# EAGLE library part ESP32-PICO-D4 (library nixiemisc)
The ESP32-PICO-D4 is a System-in-Package (SIP) module that is based on ESP32, providing complete Wi-Fi and Bluetooth functionalities. The module has a size as small as 7.0±0.1 mm×7.0±0.1 mm×0.94±0.1 mm, thus requiring minimal PCB area. The module integrates a 4-MB SPI flash
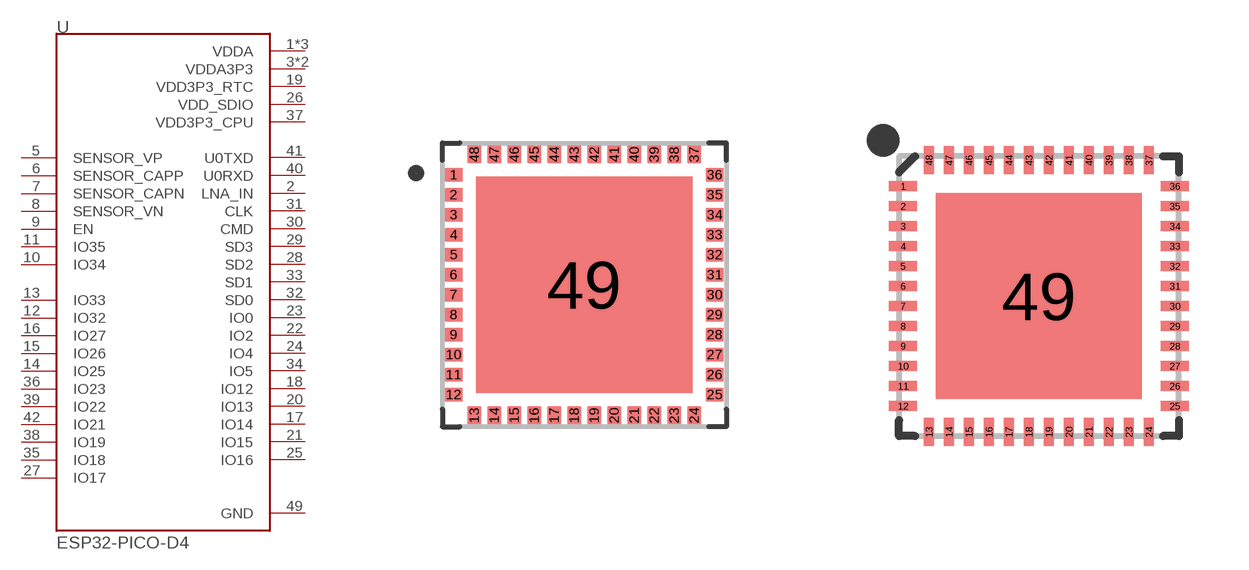
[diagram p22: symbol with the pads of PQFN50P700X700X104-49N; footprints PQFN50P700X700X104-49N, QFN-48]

Designator prefix U

## ESP32-PICO-D4 (AVAILABILITY: Unavailable; DESCRIPTION: WIFi/Bluetooth SIP; MF: Espressif Systems; MP: ESP32-PICO-D4; PACKAGE: SMD-48 Espressif Systems; PRICE: None)  [PQFN50P700X700X104-49N]
1  VDDA  pwr
2  LNA_IN
3  VDDA3P3  pwr
4  VDDA3P3  pwr
5  SENSOR_VP  in
6  SENSOR_CAPP  in
7  SENSOR_CAPN  in
8  SENSOR_VN  in
9  EN  in
10  IO34  in
11  IO35  in
12  IO32
13  IO33
14  IO25
15  IO26
16  IO27
17  IO14
18  IO12
19  VDD3P3_RTC  pwr
20  IO13
21  IO15
22  IO2
23  IO0
24  IO4
25  IO16
26  VDD_SDIO  pwr
27  IO17
28  SD2
29  SD3
30  CMD
31  CLK
32  SD0
33  SD1
34  IO5
35  IO18
36  IO23
37  VDD3P3_CPU  pwr
38  IO19
39  IO22
40  U0RXD
41  U0TXD
42  IO21
43  VDDA  pwr
46  VDDA  pwr
49  GND  pwr

## ESP32-PICO-D4QFN-48  [QFN-48]
Pads as for PQFN50P700X700X104-49N

## ESP32-PICO-D4QFN-48-7X7  [QFN48_7X7]
Pads as for PQFN50P700X700X104-49N

## Footprint PQFN50P700X700X104-49N (pad centres in mm)
smd 0.45 x 0.35: 1 -3.265,2.75; 2 -3.265,2.25; 3 -3.265,1.75; 4 -3.265,1.25; 5 -3.265,0.75; 6 -3.265,0.25; 7 -3.265,-0.25; 8 -3.265,-0.75; 9 -3.265,-1.25; 10 -3.265,-1.75; 11 -3.265,-2.25; 12 -3.265,-2.75; 25 3.265,-2.75; 26 3.265,-2.25; 27 3.265,-1.75; 28 3.265,-1.25; 29 3.265,-0.75; 30 3.265,-0.25; 31 3.265,0.25; 32 3.265,0.75; 33 3.265,1.25; 34 3.265,1.75; 35 3.265,2.25; 36 3.265,2.75
smd 0.35 x 0.45: 13 -2.75,-3.265; 14 -2.25,-3.265; 15 -1.75,-3.265; 16 -1.25,-3.265; 17 -0.75,-3.265; 18 -0.25,-3.265; 19 0.25,-3.265; 20 0.75,-3.265; 21 1.25,-3.265; 22 1.75,-3.265; 23 2.25,-3.265; 24 2.75,-3.265; 37 2.75,3.265; 38 2.25,3.265; 39 1.75,3.265; 40 1.25,3.265; 41 0.75,3.265; 42 0.25,3.265; 43 -0.25,3.265; 44 -0.75,3.265; 45 -1.25,3.265; 46 -1.75,3.265; 47 -2.25,3.265; 48 -2.75,3.265
smd 5.4 x 5.4: 49 0,0

## Footprint QFN-48 (pad centres in mm)
48-pin QFN (7x7mm, 0.5mm pitch) Used on: ATSAMD21G
smd 0.7 x 0.25: 1 -3.4,2.75; 2 -3.4,2.25; 3 -3.4,1.75; 4 -3.4,1.25; 5 -3.4,0.75; 6 -3.4,0.25; 7 -3.4,-0.25; 8 -3.4,-0.75; 9 -3.4,-1.25; 10 -3.4,-1.75; 11 -3.4,-2.25; 12 -3.4,-2.75; 25 3.4,-2.75; 26 3.4,-2.25; 27 3.4,-1.75; 28 3.4,-1.25; 29 3.4,-0.75; 30 3.4,-0.25; 31 3.4,0.25; 32 3.4,0.75; 33 3.4,1.25; 34 3.4,1.75; 35 3.4,2.25; 36 3.4,2.75
smd 0.25 x 0.7: 13 -2.75,-3.4; 14 -2.25,-3.4; 15 -1.75,-3.4; 16 -1.25,-3.4; 17 -0.75,-3.4; 18 -0.25,-3.4; 19 0.25,-3.4; 20 0.75,-3.4; 21 1.25,-3.4; 22 1.75,-3.4; 23 2.25,-3.4; 24 2.75,-3.4; 37 2.75,3.4; 38 2.25,3.4; 39 1.75,3.4; 40 1.25,3.4; 41 0.75,3.4; 42 0.25,3.4; 43 -0.25,3.4; 44 -0.75,3.4; 45 -1.25,3.4; 46 -1.75,3.4; 47 -2.25,3.4; 48 -2.75,3.4
smd 5.15 x 5.15: 49 0,0

## Footprint QFN48_7X7 (pad centres in mm)
smd 1 x 0.28: 1 -3.575,2.75; 2 -3.575,2.25; 3 -3.575,1.75; 4 -3.575,1.25; 5 -3.575,0.75; 6 -3.575,0.25; 7 -3.575,-0.25; 8 -3.575,-0.75; 9 -3.575,-1.25; 10 -3.575,-1.75; 11 -3.575,-2.25; 12 -3.575,-2.75; 25 3.575,-2.75; 26 3.575,-2.25; 27 3.575,-1.75; 28 3.575,-1.25; 29 3.575,-0.75; 30 3.575,-0.25; 31 3.575,0.25; 32 3.575,0.75; 33 3.575,1.25; 34 3.575,1.75; 35 3.575,2.25; 36 3.575,2.75
smd 0.28 x 1: 13 -2.75,-3.575; 14 -2.25,-3.575; 15 -1.75,-3.575; 16 -1.25,-3.575; 17 -0.75,-3.575; 18 -0.25,-3.575; 19 0.25,-3.575; 20 0.75,-3.575; 21 1.25,-3.575; 22 1.75,-3.575; 23 2.25,-3.575; 24 2.75,-3.575; 37 2.75,3.575; 38 2.25,3.575; 39 1.75,3.575; 40 1.25,3.575; 41 0.75,3.575; 42 0.25,3.575; 43 -0.25,3.575; 44 -0.75,3.575; 45 -1.25,3.575; 46 -1.75,3.575; 47 -2.25,3.575; 48 -2.75,3.575
smd 5.2 x 5.2: 49 0,0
